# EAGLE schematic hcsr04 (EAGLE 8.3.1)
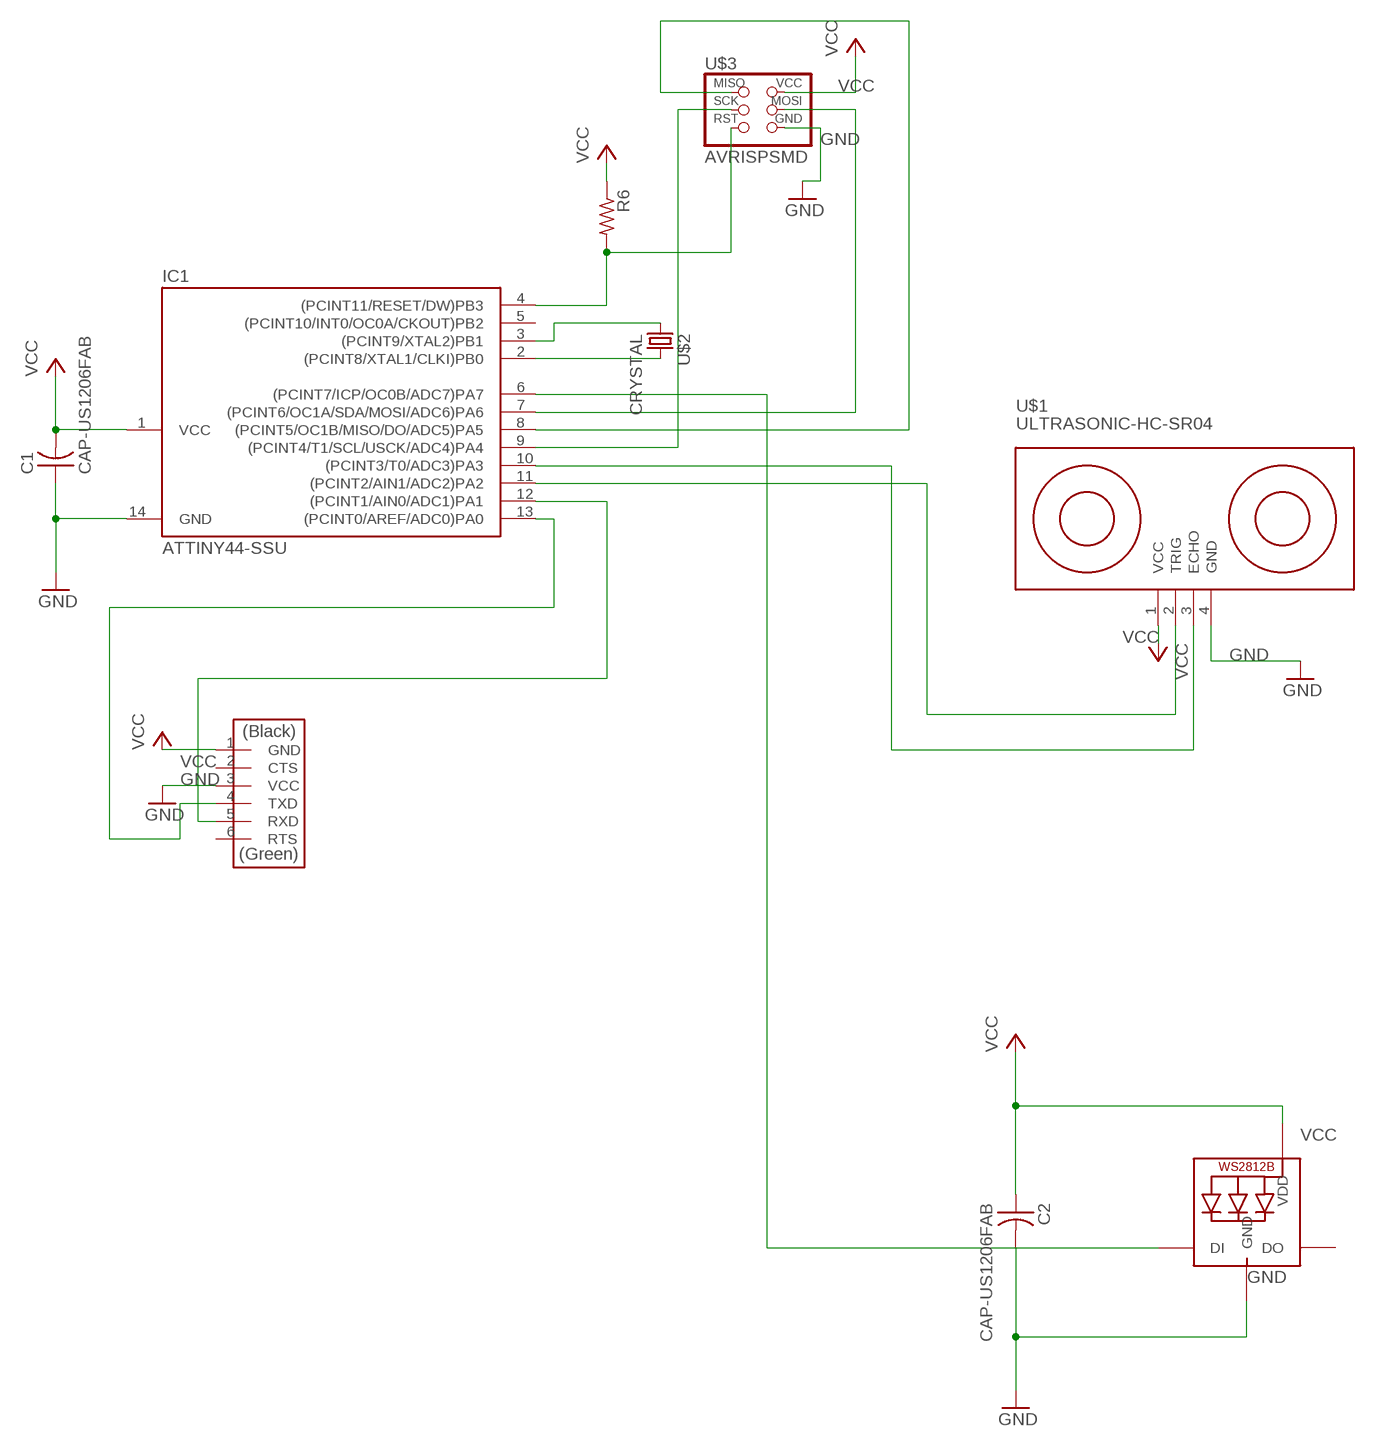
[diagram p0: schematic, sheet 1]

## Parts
C1  CAP-US1206FAB  [C1206FAB]
C2  CAP-US1206FAB  [C1206FAB]
IC1  ATTINY44-SSU  [SOIC14]
LED1  WS2812B_5050N  [WS2812B-NARROW]
R6  RES-US1206FAB  [R1206FAB]
U$1  ULTRASONIC-HC-SR04  [ULTRASONIC-HC-SR04]
U$2  CRYSTAL  [2-SMD-5X3MM]
U$3  AVRISPSMD  [2X03SMD]
U$4  FTDI-SMD-HEADER  [1X06SMD]

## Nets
GND: C1.1 C2.2 IC1.14(GND) LED1.3-GND(GND) U$1.4(GND) U$3.6(GND) U$4.3(VCC)
N$1: IC1.3((PCINT9/XTAL2)PB1) U$2.P$1
N$2: IC1.2((PCINT8/XTAL1/CLKI)PB0) U$2.P$2
N$3: IC1.11((PCINT2/AIN1/ADC2)PA2) U$1.2(TRIG)
N$4: IC1.10((PCINT3/T0/ADC3)PA3) U$1.3(ECHO)
N$5: IC1.4((PCINT11/RESET/DW)PB3) R6.2 U$3.5(RST)
N$6: IC1.7((PCINT6/OC1A/SDA/MOSI/ADC6)PA6) U$3.4(MOSI)
N$7: IC1.8((PCINT5/OC1B/MISO/DO/ADC5)PA5) U$3.1(MISO)
N$9: IC1.9((PCINT4/T1/SCL/USCK/ADC4)PA4) U$3.3(SCK)
N$11: IC1.6((PCINT7/ICP/OC0B/ADC7)PA7) LED1.4-DIN(DI)
N$13: IC1.13((PCINT0/AREF/ADC0)PA0) U$4.4(TXD)
N$14: IC1.12((PCINT1/AIN0/ADC1)PA1) U$4.5(RXD)
VCC: C1.2 C2.1 IC1.1(VCC) LED1.1-VDD(VDD) R6.1 U$1.1(VCC) U$3.2(VCC) U$4.1(GND)
Unconnected: IC1.5((PCINT10/INT0/OC0A/CKOUT)PB2) LED1.2-DOUT(DO) U$4.2(CTS) U$4.6(RTS)

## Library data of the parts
C1 C2 = fab:CAP-US
IC1 = fab:ATTINY44
LED1 = adafruit:WS2812B
R6 = fab:RES-US: Resistor (US Symbol)
U$1 = diy-modules:ULTRASONIC-HC-SR04: Ultrasonic Ranging Module HC-SR04 More details available here: http://randomnerdtutorials.com/complete-guide-for-ultrasonic-sensor-hc-sr04/ Click here to find device on ebay.com
U$2 = fab:CRYSTAL
U$3 = fab:AVRISP
U$4 = fab:FTDI-SMD-HEADER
